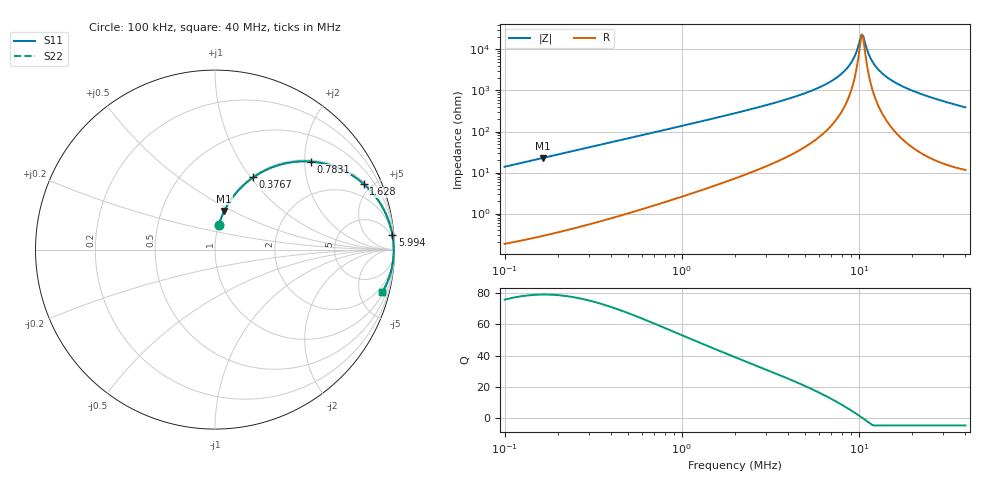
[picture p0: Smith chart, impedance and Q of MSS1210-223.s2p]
# MHz S MA R 50
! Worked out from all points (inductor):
!   263 points, 100 kHz to 40 MHz, reference 50 ohm
!   read as one part in series: L = 22 uH near 102.3 kHz
!   highest Q = 79.3 at 165.4 kHz (marker M1), where L = 21.9 uH
!   self-resonance near 10.38 MHz
!   S11 on the Smith chart (normalised r, x): 100 kHz: 1.00, +0.28; 376.7 kHz: 1.01, +1.03; 783.1 kHz: 1.04, +2.14; 1.628 MHz: 1.10, +4.50; 5.994 MHz: 2, +24; 40 MHz: 1.23, -7.77
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0.1  0.1367 81.4  0.9888 -7.9  0.9888 -7.9  0.1367 81.4
0.165384  0.2214 76.5  0.9724 -12.8  0.9724 -12.8  0.2214 76.5
0.2735188  0.3497 68.8  0.9323 -20.5  0.9323 -20.5  0.3497 68.8
0.3767286  0.4556 62.1  0.8839 -27.1  0.8839 -27.1  0.4556 62.1
0.7481253  0.7086 43.9  0.6937 -45.1  0.6937 -45.1  0.7086 43.9
0.7831364  0.7242 42.6  0.6772 -46.4  0.6772 -46.4  0.7242 42.6
1.627969  0.9061 23.7  0.4025 -64.9  0.4025 -64.9  0.9061 23.7
2  0.934 19.5  0.334 -69.0  0.334 -69.0  0.934 19.5
3.624513  0.9777 10.2  0.177 -77.7  0.177 -77.7  0.9777 10.2
5.470376  0.9898 5.6  0.09829 -81.2  0.09829 -81.2  0.9898 5.6
5.994366  0.9914 4.8  0.08311 -81.7  0.08311 -81.7  0.9914 4.8
7.364224  0.994 2.9  0.05103 -81.8  0.05103 -81.8  0.994 2.9
8.642665  0.9952 1.6  0.02755 -79.1  0.02755 -79.1  0.9952 1.6
9.47052  0.9956 0.8  0.01464 -72.1  0.01464 -72.1  0.9956 0.8
10.37767  0.9958 0.1  0.004291 -11.9  0.004291 -11.9  0.9958 0.1
10.61772  0.9958 -0.1  0.004804 29.6  0.004804 29.6  0.9958 -0.1
11.11462  0.9958 -0.5  0.009841 64.7  0.009841 64.7  0.9958 -0.5
11.90389  0.9958 -1.1  0.01924 76.7  0.01924 76.7  0.9958 -1.1
13.04413  0.9955 -1.8  0.03236 81.1  0.03236 81.1  0.9955 -1.8
14.96251  0.9947 -3.0  0.05274 82.7  0.05274 82.7  0.9947 -3.0
21.57291  0.9894 -6.5  0.1128 81.4  0.1128 81.4  0.9894 -6.5
40  0.9615 -14.3  0.2475 74.0  0.2475 74.0  0.9615 -14.3
